//{{V2}}
FUNCTION FC14
TITLE=


AUTHOR:INA
FAMILY:SDO
NAME:WrtUInt8
VERSION:00.01


VAR_INPUT
       IN0:BYTE
       IN1:DWORD
       IN2:DWORD
       IN3:BYTE
END_VAR

VAR_OUTPUT
       RET_VAL:BOOL
       OUT4:BOOL
       OUT5:DINT
END_VAR

VAR_IN_OUT
END_VAR

VAR_TEMP
       TEMP6:BOOL
       TEMP7:DWORD
       TEMP8:WORD
       TEMP9:BYTE
END_VAR
BEGIN

NETWORK
TITLE=
//{{a}}

       R    #RET_VAL
       R    #OUT4
       L    0
       T    #OUT5
       L    #IN3
       T    #TEMP9
M000  :NOP  0
       CALL SFC219
         Request:=TRUE
         Slot_Master:=B#16#00
         NodeID:=#IN0
         Transfertyp:=B#16#61
         Index:=#IN1
         Subindex:=#IN2
         CanOpenError:=#TEMP7
         RetVal:=#TEMP8
         Busy:=#TEMP6
         DataBuffer:=P#L 8.0 BYTE 1
       L    1
       U    #TEMP6
       SPB  M000
       S    #RET_VAL
       L    W#16#F021
       L    #TEMP8
       <I
       SPBN M001
       L    W#16#F028
       L    #TEMP8
       >I
       SPB  M002
       L    0
       L    #TEMP7
       <>D
       SPB  M003
M001  :NOP  0
       R    #OUT4
       SPA  M004
M003  :NOP  0
       S    #OUT4
       L    #TEMP7
       TAD
       T    #OUT5
       SPA  M004
M002  :NOP  0
       S    #OUT4
       L    0
       T    #OUT5
       L    #TEMP8
       T    #OUT5
M004  :NOP  0
END_FUNCTION
